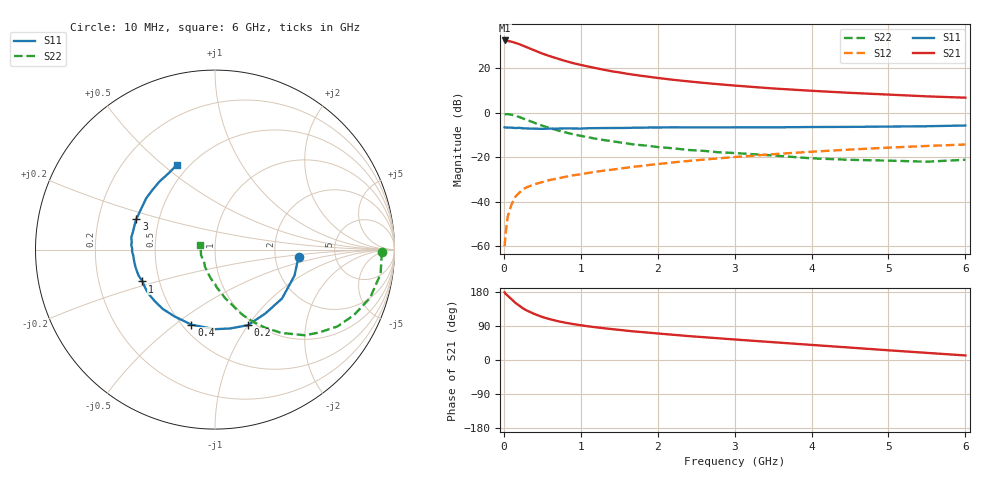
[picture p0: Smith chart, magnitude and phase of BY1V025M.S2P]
! SIEMENS Small Signal Semiconductors
! BFY420
! Si NPN RF SIEGET Grounded Emitter Transistor in MICRO-X
! VCE = 1 V  IC = 25 mA
! Common Emitter S-Parameters:  October  1996
# GHz  S  MA  R  50
!  f  S11  S21  S12  S22
! GHz  MAG  ANG  MAG  ANG  MAG  ANG  MAG  ANG
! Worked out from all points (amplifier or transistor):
!   36 points, 10 MHz to 6 GHz, reference 50 ohm
!   highest |S21| = 32.5 dB at 10 MHz (marker M1)
!   |S21| within 3 dB of that: start of sweep to 294.4 MHz
!   unconditionally stable (mu >= 1): start of sweep to 12.15 MHz; 1.563 GHz to end of sweep
!   at 250 MHz: K = 0.35, MSG = 32.3 dB, |S12| = -34.4 dB
!   at 1.4 GHz: K = 0.97, MSG = 22.2 dB, |S12| = -25.6 dB
!   at 6 GHz: K = 1.09, MAG = 8.7 dB, |S12| = -14.3 dB
!   S11 on the Smith chart (normalised r, x): 10 MHz: 2.75, -0.27; 200 MHz: 0.93, -1.00; 400 MHz: 0.55, -0.57; 1 GHz: 0.40, -0.18; 3 GHz: 0.37, +0.16; 6 GHz: 0.43, +0.56
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0.01  0.4704 -4.7  42.3 178.7  0.001 109.4  0.9284 -0.8
0.02  0.4647 -7.8  42.08 175.3  0.0017 90.3  0.9288 -2.7
0.1  0.4623 -36.1  39.73 160.5  0.0087 78.3  0.905 -17.3
0.15  0.4533 -51.9  37.27 150.8  0.0129 70.7  0.8555 -25.3
0.2  0.4591 -66.6  34.95 143.5  0.0159 67.8  0.8047 -32.2
0.25  0.4475 -79.1  32.19 136.2  0.019 64.4  0.7417 -38.5
0.3  0.4434 -90.1  29.67 130.4  0.0212 62.0  0.6921 -43.6
0.4  0.4385 -107.5  25.21 121.2  0.0247 57.9  0.5921 -51.6
0.5  0.4353 -121.3  21.43 113.4  0.0276 56.3  0.512 -57.7
0.6  0.4406 -131.4  18.7 107.6  0.0308 55.5  0.4511 -62.4
0.7  0.4415 -139.6  16.5 102.5  0.0333 55.6  0.403 -66.4
0.8  0.4447 -146.1  14.6 98.4  0.0363 55.0  0.3621 -69.7
1  0.4414 -156.3  11.92 91.7  0.0414 55.8  0.3032 -74.7
1.1  0.4497 -161.1  10.94 88.8  0.0443 56.2  0.2807 -77.7
1.4  0.4547 -171.1  8.598 81.6  0.0524 56.4  0.2301 -83.9
1.6  0.4568 -176.1  7.546 77.2  0.0583 55.7  0.2042 -88.3
2.2  0.4714 171.6  5.516 66.6  0.0764 53.8  0.159 -99.1
3  0.4701 158.8  4.092 54.1  0.1012 49.2  0.1245 -111.7
3.5  0.4701 150.6  3.522 47.0  0.117 45.7  0.1095 -120.8
4.5  0.4815 136.5  2.807 32.8  0.1487 36.7  0.0875 -139.3
5.5  0.498 121.1  2.339 18.8  0.1794 26.6  0.0793 -176.3
6  0.5171 114.4  2.184 12.0  0.1932 21.5  0.0878 164.6
